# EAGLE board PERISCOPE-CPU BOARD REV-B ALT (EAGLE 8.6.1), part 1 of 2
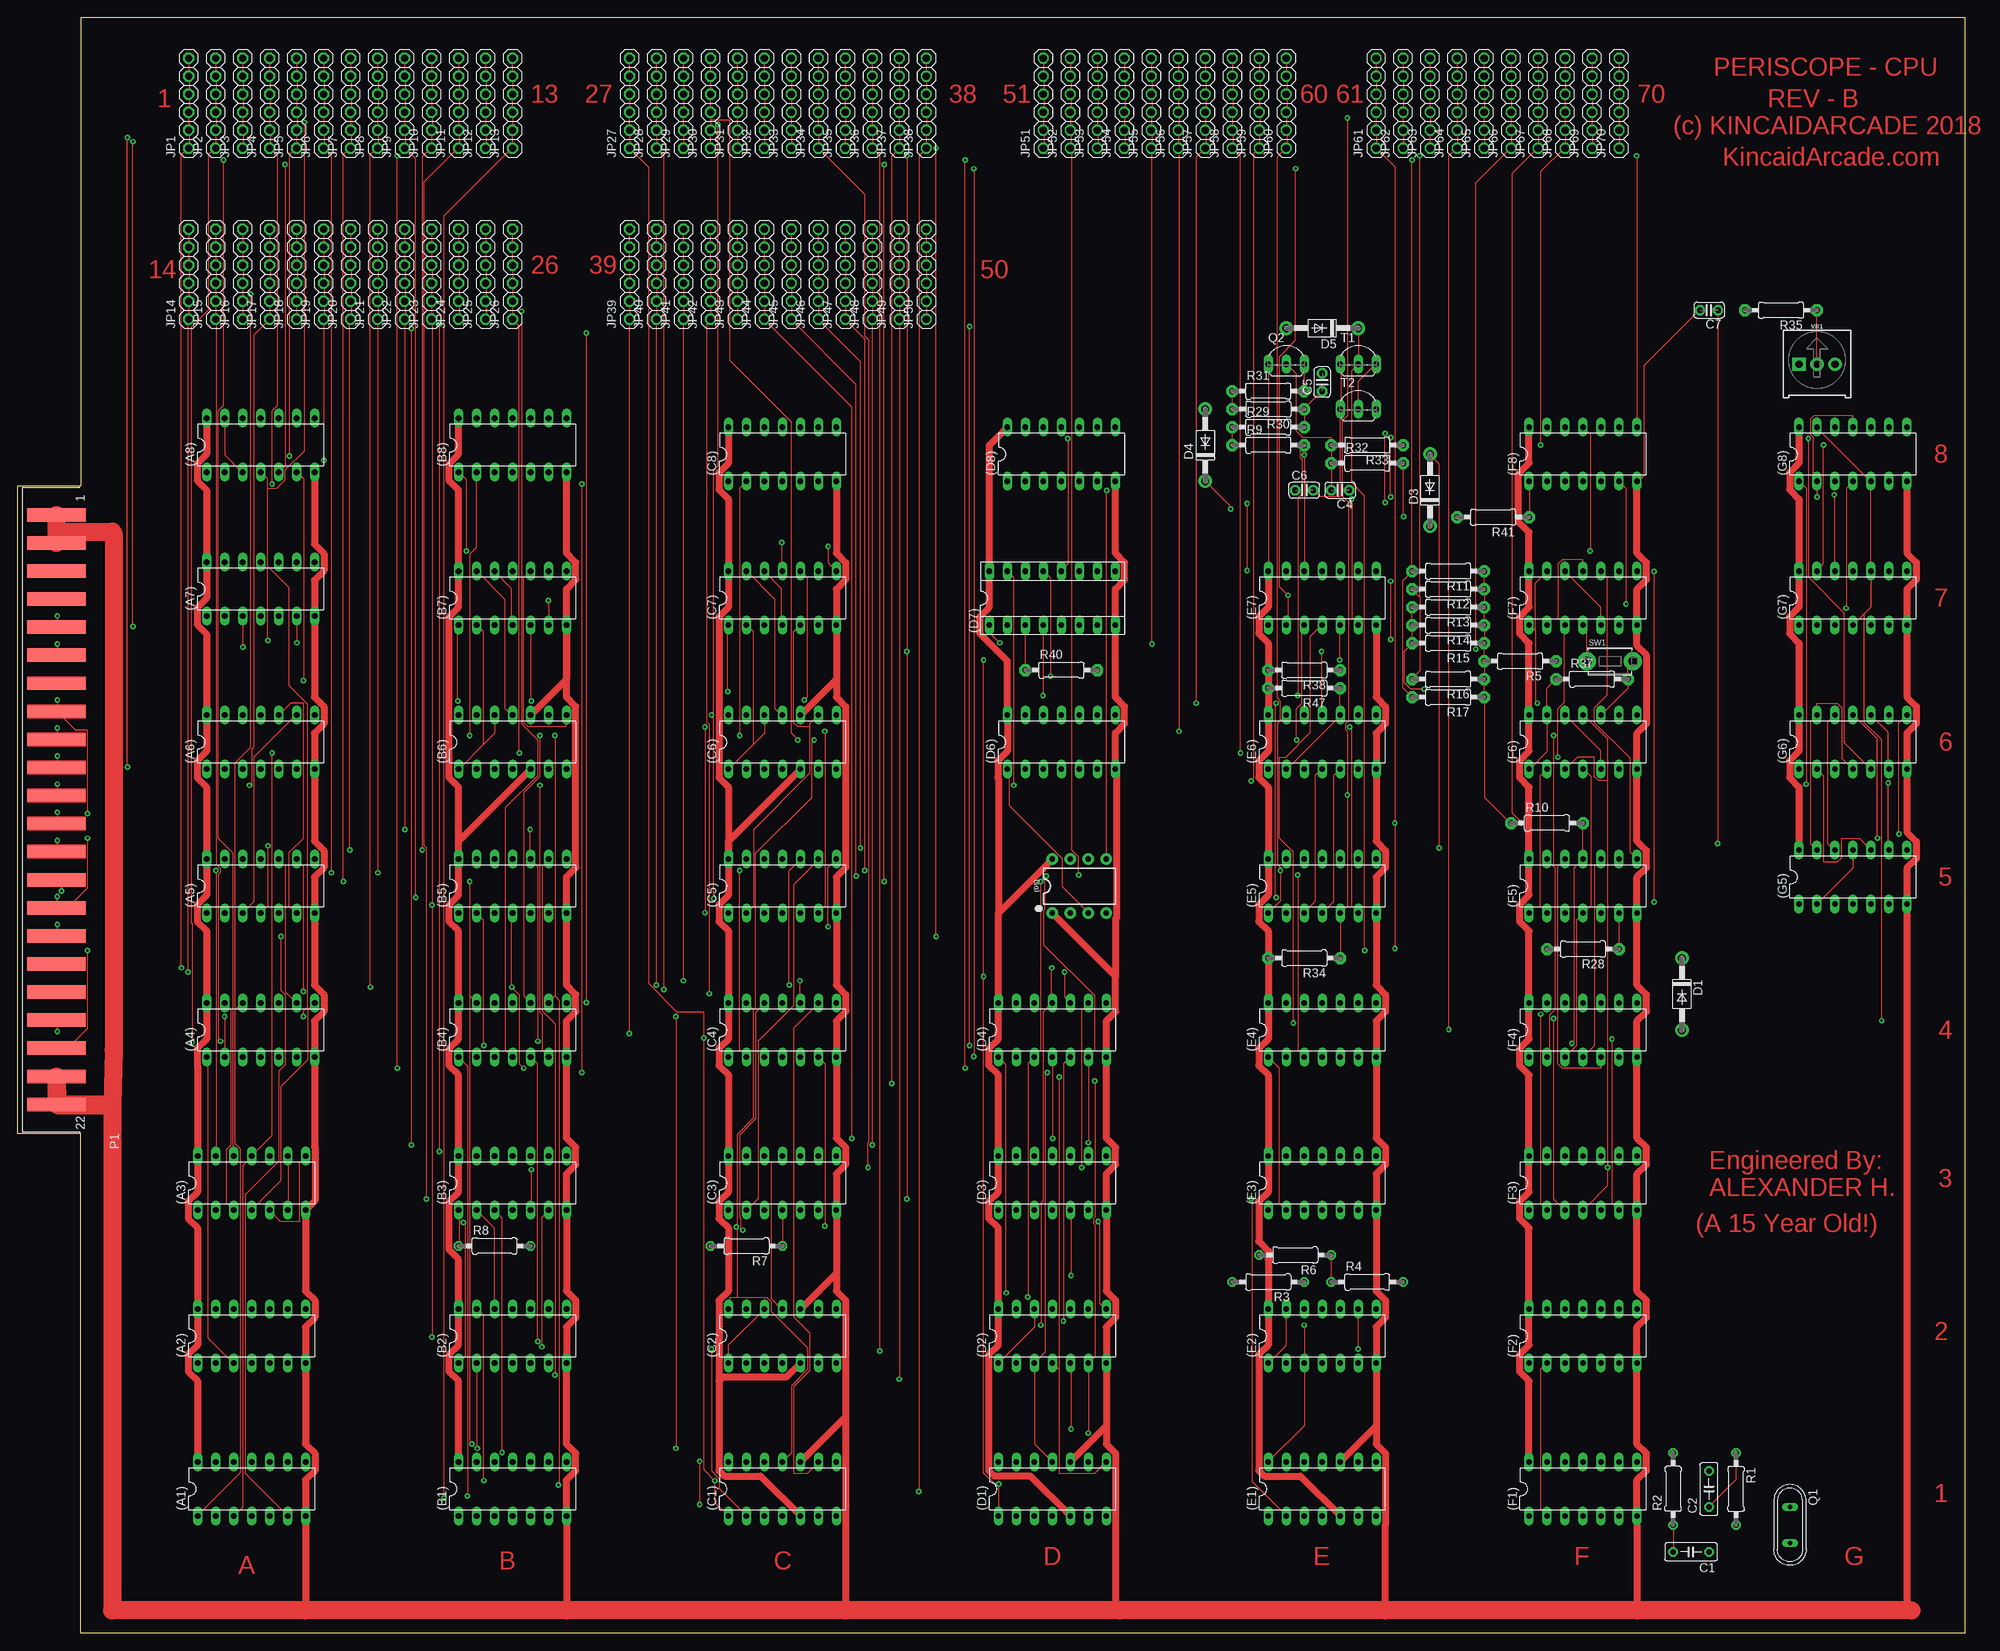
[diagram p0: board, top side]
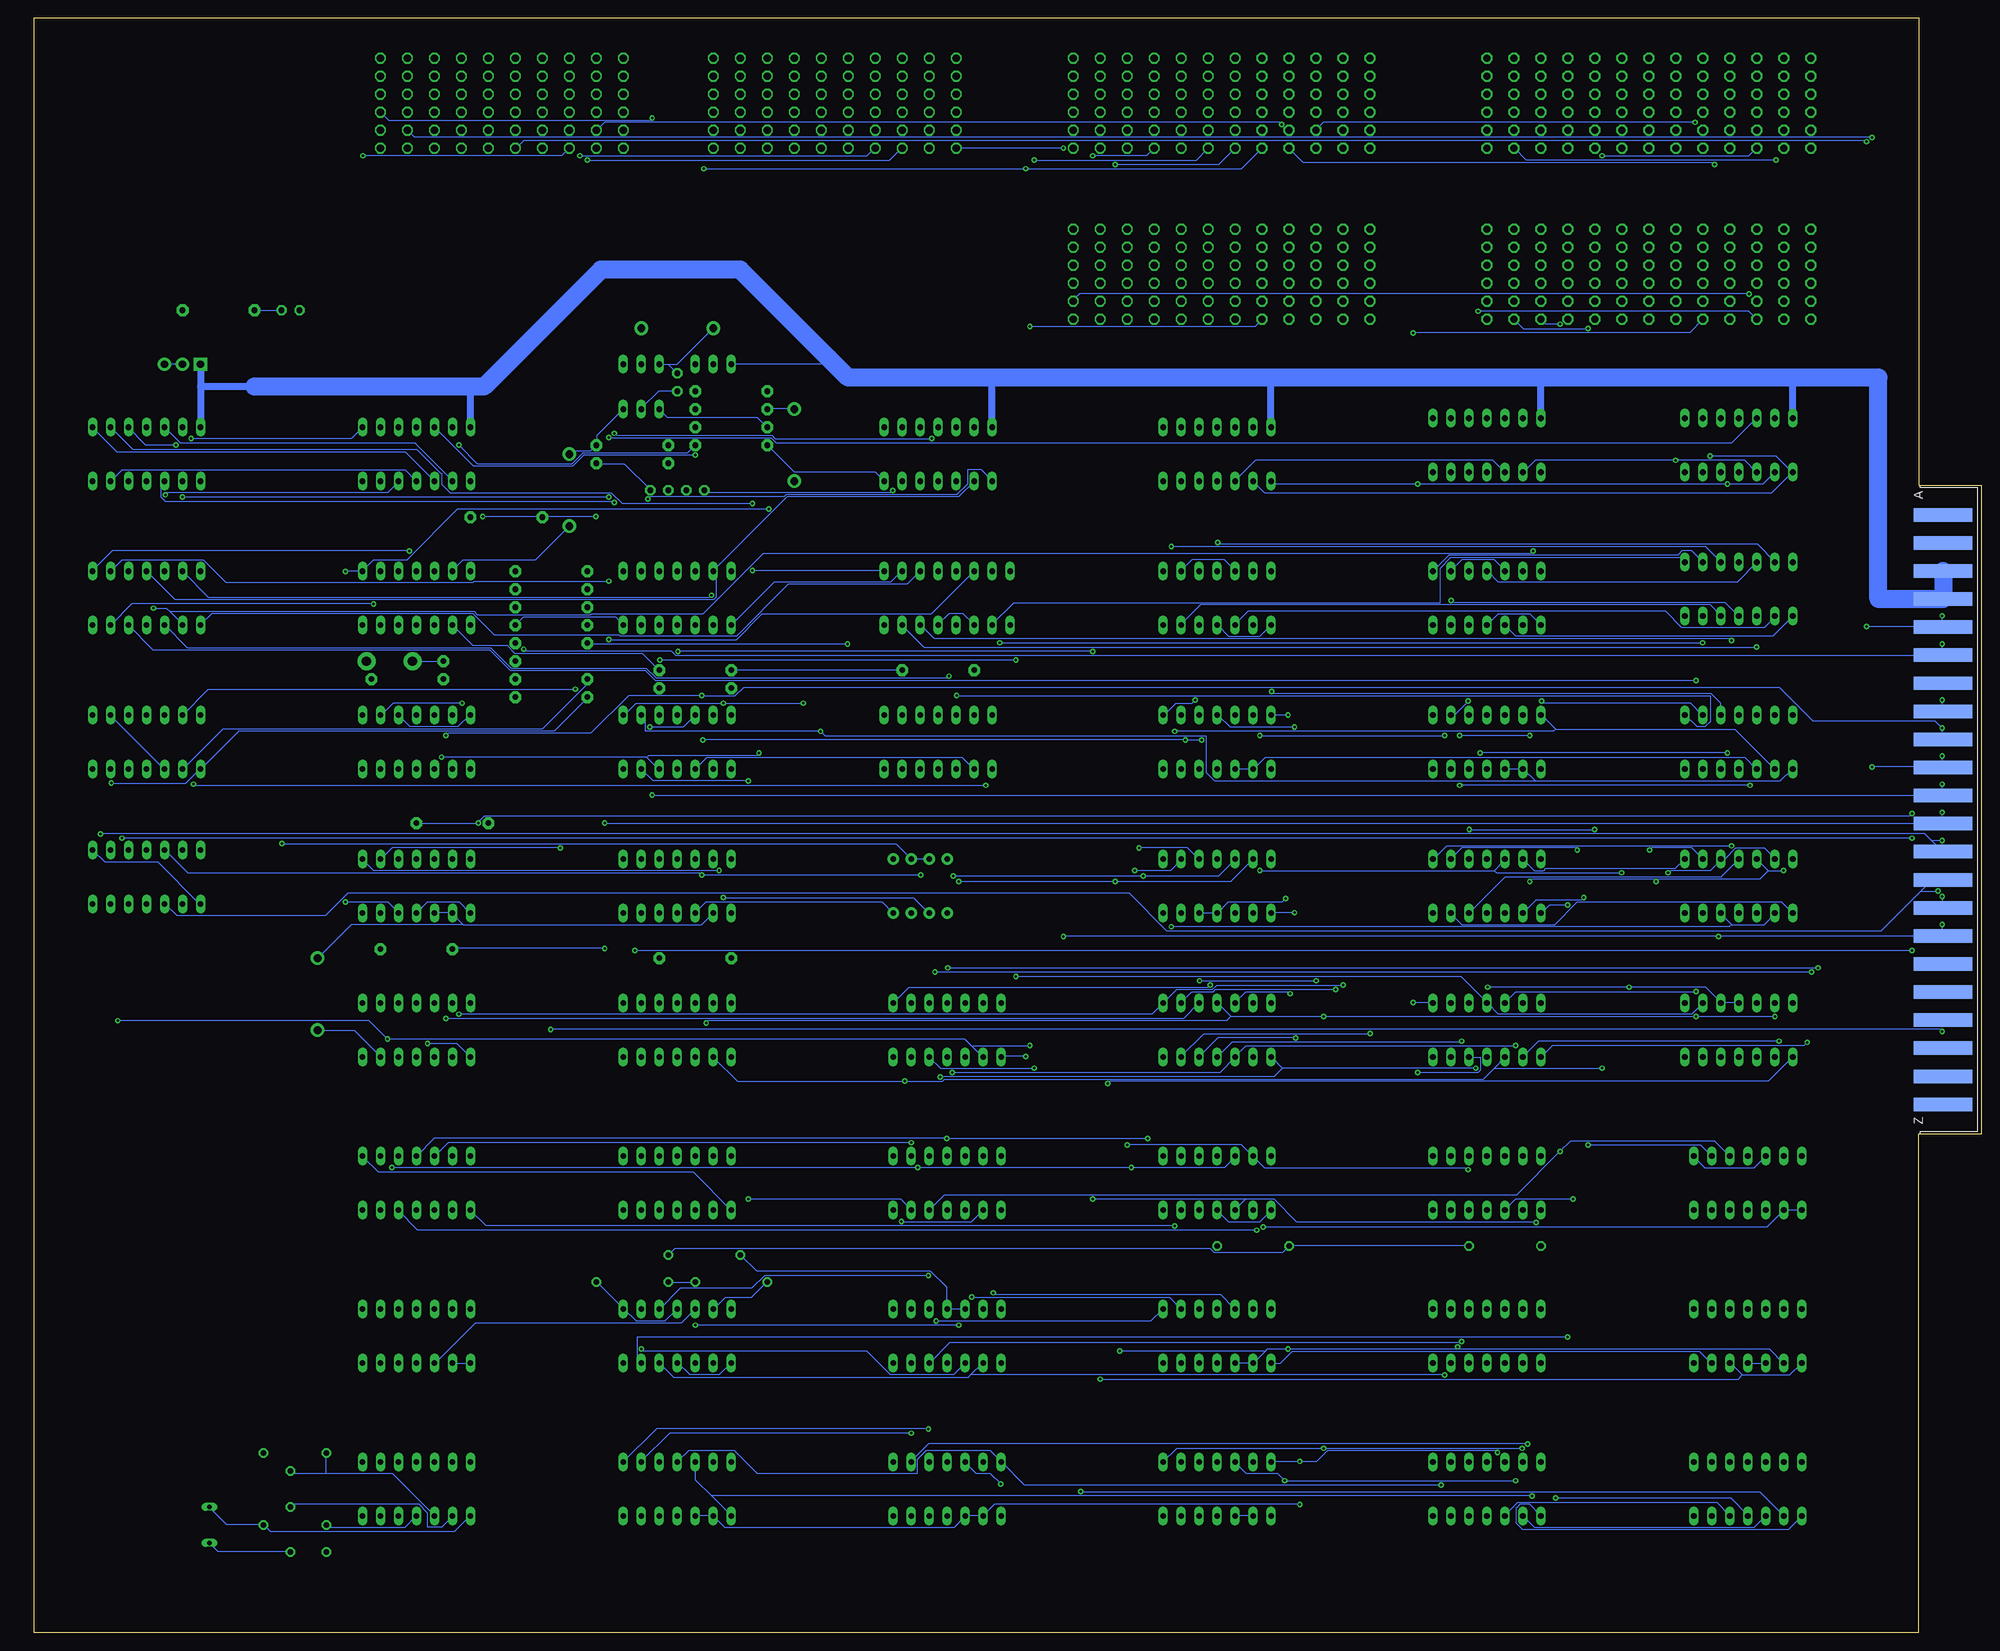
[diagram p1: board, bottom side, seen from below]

Size 274.96 x 227.97 mm. Coordinates in mm from the lower left corner, seen from the top.
Outline: 8.89,0 8.89,70.48 0,70.48 0,161.93 8.89,161.93 8.89,227.97 274.96,227.97 274.96,0 8.89,0
Copper layers (1*16): Top 0.035mm / dielectric 1.5mm / Bottom 0.035mm
Design rules "default": minimum track width 6mil, minimum drill 0.35mm, track to track 6mil, track to pad 6mil, pad to pad 6mil, via to via 6mil, smd to smd 6mil, copper to edge 40mil, drill to drill 6mil, minimum pad ring 10mil, minimum via ring 8mil, stop-mask expansion 4mil, vias tented up to drill 0mil, thermal gap 10mil

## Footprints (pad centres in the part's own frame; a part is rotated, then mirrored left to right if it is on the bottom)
DIL14 = drill 0.813 long: 1 -7.62,-3.81; 2 -5.08,-3.81; 3 -2.54,-3.81; 4 0,-3.81; 5 2.54,-3.81; 6 5.08,-3.81; 7 7.62,-3.81; 8 7.62,3.81; 9 5.08,3.81; 10 2.54,3.81; 11 0,3.81; 12 -2.54,3.81; 13 -5.08,3.81; 14 -7.62,3.81
DIP08 = drill 0.813 pad 1.626: 1 -3.81,-3.81; 2 -1.27,-3.81; 3 1.27,-3.81; 4 3.81,-3.81; 5 3.81,3.81; 6 1.27,3.81; 7 -1.27,3.81; 8 -3.81,3.81
SOCKET-16 = drill 0.813 long: 1 -8.89,-3.81; 2 -6.35,-3.81; 3 -3.81,-3.81; 4 -1.27,-3.81; 5 1.27,-3.81; 6 3.81,-3.81; 7 6.35,-3.81; 8 8.89,-3.81; 9 8.89,3.81; 10 6.35,3.81; 11 3.81,3.81; 12 1.27,3.81; 13 -1.27,3.81; 14 -3.81,3.81; 15 -6.35,3.81; 16 -8.89,3.81
C050-025X075 = drill 0.813 octagon: 1 -2.54,0; 2 2.54,0
C025-024X044 = drill 0.813 pad 1.422 octagon: 1 -1.27,0; 2 1.27,0
DO41-10 = drill 1.118 pad 1.93: A 5.08,0; C -5.08,0
1X06 = drill 1.016 octagon: 1 -6.35,0; 2 -3.81,0; 3 -1.27,0; 4 1.27,0; 5 3.81,0; 6 6.35,0
44PINEDGE = smd 1.905 x 8.255: 1 -41.605,4.826; 2 -37.643,4.826; 3 -33.68,4.826; 4 -29.718,4.826; 5 -25.756,4.826; 6 -21.793,4.826; 7 -17.831,4.826; 8 -13.868,4.826; 9 -9.906,4.826; 10 -5.944,4.826; 11 -1.981,4.826; 12 1.981,4.826; 13 5.944,4.826; 14 9.906,4.826; 15 13.868,4.826; 16 17.831,4.826; 17 21.793,4.826; 18 25.756,4.826; 19 29.718,4.826; 20 33.68,4.826; 21 37.643,4.826; 22 41.605,4.826 | smd 1.905 x 8.255 bottom: A -41.605,4.826; B -37.643,4.826; C -33.68,4.826; D -29.718,4.826; E -25.756,4.826; F -21.793,4.826; H -17.831,4.826; J -13.868,4.826; K -9.906,4.826; L -5.944,4.826; M -1.981,4.826; N 1.981,4.826; P 5.944,4.826; R 9.906,4.826; S 13.868,4.826; T 17.831,4.826; U 21.793,4.826; V 25.756,4.826; W 29.718,4.826; X 33.68,4.826; Y 37.643,4.826; Z 41.605,4.826
QS = drill 0.61 long: 1 -2.54,0; 2 2.54,0
TO92-EBC-OVAL = drill 0.813 long: B 0,-1.27; C 2.54,-1.27; E -2.54,-1.27
0207/10 = drill 0.813 octagon: 1 -5.08,0; 2 5.08,0
0207/10' = drill 0.813 pad 1.676 octagon: 1 -5.08,0; 2 5.08,0
TACT_PANA-EVQ = drill 1.3 pad 2.54: P$1 -3.25,0; P$2 3.25,0
TRIMPOT-PTH-3386U = drill 1.016 pad 1.88 square: 1 -2.54,-0.015 | drill 1.016 pad 1.88: 2 0,-0.015; 3 2.54,-0.015

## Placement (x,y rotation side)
(A1)  7404N  [DIL14]  33.02,20.32 0 top
(A2)  7402N  [DIL14]  33.02,41.91 0 top
(A3)  7400N  [DIL14]  33.02,63.5 0 top
(A4)  7410N  [DIL14]  34.29,85.09 0 top
(A5)  74S08N  [DIL14]  34.29,105.41 0 top
(A6)  7432N  [DIL14]  34.29,125.73 0 top
(A7)  7432N  [DIL14]  34.29,147.32 0 top
(A8)  74LS27N  [DIL14]  34.29,167.64 0 top
(B1)  7486N  [DIL14]  69.85,20.32 0 top
(B2)  7410N  [DIL14]  69.85,41.91 0 top
(B3)  74S74N  [DIL14]  69.85,63.5 0 top
(B4)  7404N  [DIL14]  69.85,85.09 0 top
(B5)  74LS21N  [DIL14]  69.85,105.41 0 top
(B6)  74LS93N  [DIL14]  69.85,125.73 0 top
(B7)  74S08N  [DIL14]  69.85,146.05 0 top
(B8)  7402N  [DIL14]  69.85,167.64 0 top
(C1)  74LS93N  [DIL14]  107.95,20.32 0 top
(C2)  74LS93N  [DIL14]  107.95,41.91 0 top
(C3)  74107N  [DIL14]  107.95,63.5 0 top
(C4)  7404N  [DIL14]  107.95,85.09 0 top
(C5)  74LS21N  [DIL14]  107.95,105.41 0 top
(C6)  74LS93N  [DIL14]  107.95,125.73 0 top
(C7)  74S08N  [DIL14]  107.95,146.05 0 top
(C8)  7400N  [DIL14]  107.95,166.37 0 top
(D1)  74LS93N  [DIL14]  146.05,20.32 0 top
(D2)  7430N  [DIL14]  146.05,41.91 0 top
(D3)  74LS74N  [DIL14]  146.05,63.5 0 top
(D4)  7404N  [DIL14]  146.05,85.09 0 top
(D5)  555  [DIP08]  149.86,105.41 0 top
(D6)  7404N  [DIL14]  147.32,125.73 0 top
(D7)  7448  [SOCKET-16]  146.05,146.05 0 top
(D8)  7404N  [DIL14]  147.32,166.37 0 top
(E1)  74LS93N  [DIL14]  184.15,20.32 0 top
(E2)  74LS107N  [DIL14]  184.15,41.91 0 top
(E3)  7404N  [DIL14]  184.15,63.5 0 top
(E4)  74S08N  [DIL14]  184.15,85.09 0 top
(E5)  74S08N  [DIL14]  184.15,105.41 0 top
(E6)  74S74N  [DIL14]  184.15,125.73 0 top
(E7)  7410N  [DIL14]  184.15,146.05 0 top
(F1)  7404N  [DIL14]  220.98,20.32 0 top
(F2)  7400N  [DIL14]  220.98,41.91 0 top
(F3)  7430N  [DIL14]  220.98,63.5 0 top
(F4)  7432N  [DIL14]  220.98,85.09 0 top
(F5)  7404N  [DIL14]  220.98,105.41 0 top
(F6)  74S74N  [DIL14]  220.98,125.73 0 top
(F7)  74S74N  [DIL14]  220.98,146.05 0 top
(F8)  7430N  [DIL14]  220.98,166.37 0 top
(G5)  7432N  [DIL14]  259.08,106.68 0 top
(G6)  7432N  [DIL14]  259.08,125.73 0 top
(G7)  7410N  [DIL14]  259.08,146.05 0 top
(G8)  7410N  [DIL14]  259.08,166.37 0 top
C1  100pf  [C050-025X075]  236.22,11.43 180 top
C2  .1uf  [C050-025X075]  238.76,20.32 90 top
C4  .1uf  [C025-024X044]  186.69,161.29 180 top
C5  .1uf  [C025-024X044]  184.15,176.53 90 top
C6  .01uf  [C025-024X044]  181.61,161.29 0 top
C7  100uf  [C025-024X044]  238.76,186.69 180 top
D1  1N914  [DO41-10]  234.95,90.17 270 top
D3  1N4004  [DO41-10]  199.39,161.29 90 top
D4  1N914  [DO41-10]  167.64,167.64 90 top
D5  1N914  [DO41-10]  184.15,184.15 180 top
JP1  [1X06]  24.13,215.9 90 top
JP2  [1X06]  27.94,215.9 90 top
JP3  [1X06]  31.75,215.9 90 top
JP4  [1X06]  35.56,215.9 90 top
JP5  [1X06]  39.37,215.9 90 top
JP6  [1X06]  43.18,215.9 90 top
JP7  [1X06]  46.99,215.9 90 top
JP8  [1X06]  50.8,215.9 90 top
JP9  [1X06]  54.61,215.9 90 top
JP10  [1X06]  58.42,215.9 90 top
JP11  [1X06]  62.23,215.9 90 top
JP12  [1X06]  66.04,215.9 90 top
JP13  [1X06]  69.85,215.9 90 top
JP14  [1X06]  24.13,191.77 90 top
JP15  [1X06]  27.94,191.77 90 top
JP16  [1X06]  31.75,191.77 90 top
JP17  [1X06]  35.56,191.77 90 top
JP18  [1X06]  39.37,191.77 90 top
JP19  [1X06]  43.18,191.77 90 top
JP20  [1X06]  46.99,191.77 90 top
JP21  [1X06]  50.8,191.77 90 top
JP22  [1X06]  54.61,191.77 90 top
JP23  [1X06]  58.42,191.77 90 top
JP24  [1X06]  62.23,191.77 90 top
JP25  [1X06]  66.04,191.77 90 top
JP26  [1X06]  69.85,191.77 90 top
JP27  [1X06]  86.36,215.9 90 top
JP28  [1X06]  90.17,215.9 90 top
JP29  [1X06]  93.98,215.9 90 top
JP30  [1X06]  97.79,215.9 90 top
JP31  [1X06]  101.6,215.9 90 top
JP32  [1X06]  105.41,215.9 90 top
JP33  [1X06]  109.22,215.9 90 top
JP34  [1X06]  113.03,215.9 90 top
JP35  [1X06]  116.84,215.9 90 top
JP36  [1X06]  120.65,215.9 90 top
JP37  [1X06]  124.46,215.9 90 top
JP38  [1X06]  128.27,215.9 90 top
JP39  [1X06]  86.36,191.77 90 top
JP40  [1X06]  90.17,191.77 90 top
JP41  [1X06]  93.98,191.77 90 top
JP42  [1X06]  97.79,191.77 90 top
JP43  [1X06]  101.6,191.77 90 top
JP44  [1X06]  105.41,191.77 90 top
JP45  [1X06]  109.22,191.77 90 top
JP46  [1X06]  113.03,191.77 90 top
JP47  [1X06]  116.84,191.77 90 top
JP48  [1X06]  120.65,191.77 90 top
JP49  [1X06]  124.46,191.77 90 top
JP50  [1X06]  128.27,191.77 90 top
JP51  [1X06]  144.78,215.9 90 top
JP52  [1X06]  148.59,215.9 90 top
JP53  [1X06]  152.4,215.9 90 top
JP54  [1X06]  156.21,215.9 90 top
JP55  [1X06]  160.02,215.9 90 top
JP56  [1X06]  163.83,215.9 90 top
JP57  [1X06]  167.64,215.9 90 top
JP58  [1X06]  171.45,215.9 90 top
JP59  [1X06]  175.26,215.9 90 top
JP60  [1X06]  179.07,215.9 90 top
JP61  [1X06]  191.77,215.9 90 top
JP62  [1X06]  195.58,215.9 90 top
JP63  [1X06]  199.39,215.9 90 top
JP64  [1X06]  203.2,215.9 90 top
JP65  [1X06]  207.01,215.9 90 top
JP66  [1X06]  210.82,215.9 90 top
JP67  [1X06]  214.63,215.9 90 top
JP68  [1X06]  218.44,215.9 90 top
JP69  [1X06]  222.25,215.9 90 top
JP70  [1X06]  226.06,215.9 90 top
P1  44PINEDGE  [44PINEDGE]  0.63,116.2 270 top
Q1  14.13813  [QS]  250.19,15.24 270 top
Q2  2N2907  [TO92-EBC-OVAL]  179.07,180.34 0 top
R1  330  [0207/10]  242.57,20.32 270 top
R2  330  [0207/10]  233.68,20.32 90 top
R3  1K  [0207/10]  176.53,49.53 180 top
R4  1K  [0207/10]  190.5,49.53 0 top
R5  1k  [0207/10']  212.09,137.16 180 top
R6  10k  [0207/10]  180.34,53.34 180 top
R7  1K  [0207/10]  102.87,54.61 180 top
R8  1K  [0207/10]  67.31,54.61 0 top
R9  1k  [0207/10']  176.53,167.64 0 top
R10  1k  [0207/10']  215.9,114.3 0 top
R11  1K  [0207/10']  201.93,149.86 180 top
R12  1K  [0207/10']  201.93,147.32 180 top
R13  1K  [0207/10']  201.93,144.78 180 top
R14  1K  [0207/10']  201.93,142.24 180 top
R15  1K  [0207/10']  201.93,139.7 180 top
R16  1K  [0207/10']  201.93,134.62 180 top
R17  1K  [0207/10']  201.93,132.08 180 top
R28  220  [0207/10']  220.98,96.52 180 top
R29  100  [0207/10']  176.53,170.18 0 top
R30  100  [0207/10']  176.53,172.72 180 top
R31  220  [0207/10']  176.53,175.26 0 top
R32  100  [0207/10']  190.5,165.1 0 top
R33  330  [0207/10']  190.5,167.64 180 top
R34  1K  [0207/10']  181.61,95.25 180 top
R35  220k  [0207/10']  248.92,186.69 180 top
R37  10k  [0207/10']  222.25,134.62 0 top
R38  10k  [0207/10']  181.61,135.89 180 top
R40  1K  [0207/10']  147.32,135.89 0 top
R41  1k  [0207/10']  208.28,157.48 180 top
R47  1K  [0207/10']  181.61,133.35 180 top
SW1  [TACT_PANA-EVQ]  224.79,137.16 0 top
T1  2N2222  [TO92-EBC-OVAL]  189.23,180.34 0 top
T2  2N2222  [TO92-EBC-OVAL]  189.23,173.99 0 top
VR1  1 meg  [TRIMPOT-PTH-3386U]  254,179.07 0 top

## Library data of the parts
(A1) (A2) (A3) (A4) (A5) (A6) (A7) (A8) (B1) (B2) (B3) (B4) (B5) (B6) (B7) (B8) (C1) (C2) (C3) (C4) (C5) (C6) (C7) (C8) (D1) (D2) (D3) (D4) (D6) (D8) (E1) (E2) (E3) (E4) (E5) (E6) (E7) (F1) (F2) (F3) (F4) (F5) (F6) (F7) (F8) (G5) (G6) (G7) (G8) = 74xx-us
(D5) = SparkFun-IC-Special-Function; PROD_ID: IC-09173; PROD_ID_ALT: IC-09173
(D7) = ic-package
C1 C2 R1-R4 R6-R8 = rcl
C4-C7 D1 D3-D5 JP1-JP70 Q2 R5 R9-R17 R28-R35 R37 R38 R40 R41 R47 SW1 T1 T2 = adafruit
P1 = edge-156
Q1 = special
VR1 = SparkFun-Resistors; PROD_ID: RES-09730; SF_SKU: COM-09806

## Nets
1H: (B4).1 (E1).1 (E1).12 JP2.1 JP2.2 JP2.3 JP2.4 JP2.5 JP2.6
1PSTART: (E5).5 JP70.1 JP70.2 JP70.3 JP70.4 JP70.5 JP70.6 P1.11 P1.M R34.1
1V: (B2).13 (C1).1 (C1).12 (C4).5 JP27.1 JP27.2 JP27.3 JP27.4 JP27.5 JP27.6
2H: (B4).3 (D2).6 (E1).9 (E4).2 JP3.1 JP3.2 JP3.3 JP3.4 JP3.5 JP3.6
2V: (C1).9 (C4).9 JP28.1 JP28.2 JP28.3 JP28.4 JP28.5 JP28.6
4H: (A8).2 (B4).5 (C8).1 (D2).5 (E1).8 JP4.1 JP4.2 JP4.3 JP4.4 JP4.5 JP4.6
4V: (A4).2 (A8).4 (B2).2 (C1).8 (C4).11 (E7).4 JP29.1 JP29.2 JP29.3 JP29.4 JP29.5 JP29.6
5V: R3.1 R4.1 R6.1 R7.2 R8.2
8H: (A8).1 (B4).9 (C8).2 (D1).14 (E1).11 JP5.1 JP5.2 JP5.3 JP5.4 JP5.5 JP5.6
8V: (A3).1 (A3).2 (A8).5 (C1).11 (C2).14 (C4).13 (E7).3 JP30.1 JP30.2 JP30.3 JP30.4 JP30.5 JP30.6
16H: (A4).9 (A5).10 (A5).13 (B4).11 (D1).1 (D1).12 (E7).5 JP6.1 JP6.2 JP6.3 JP6.4 JP6.5 JP6.6
16V: (A2).6 (C2).1 (C2).12 (D4).1 (E7).2 (G7).13 (G8).10 JP31.1 JP31.2 JP31.3 JP31.4 JP31.5 JP31.6
32H: (A3).13 (A5).12 (B4).13 (D1).9 JP7.1 JP7.2 JP7.3 JP7.4 JP7.5 JP7.6
32V: (C2).9 (C5).13 (D4).3 JP32.1 JP32.2 JP32.3 JP32.4 JP32.5 JP32.6
64H: (A4).10 (A4).11 (B5).4 (C4).1 (D1).8 (D2).4 JP8.1 JP8.2 JP8.3 JP8.4 JP8.5 JP8.6
64V: (C2).8 (D4).5 JP33.1 JP33.2 JP33.3 JP33.4 JP33.5 JP33.6
128H: (B5).2 (C4).3 (D1).11 (D2).3 (E2).9 JP9.1 JP9.2 JP9.3 JP9.4 JP9.5 JP9.6
128V: (C2).11 (C3).12 (D4).9 (F3).4 (F6).3 (F6).11 JP34.1 JP34.2 JP34.3 JP34.4 JP34.5 JP34.6
256H: (B5).9 (D2).2 (E2).5 JP10.1 JP10.2 JP10.3 JP10.4 JP10.5 JP10.6
256V: (B2).1 (C3).3 (E6).11 JP35.1 JP35.2 JP35.3 JP35.4 JP35.5 JP35.6
512H: (D2).1 (D2).11 (D2).12 R6.2
/1H: (B4).2 JP15.1 JP15.2 JP15.3 JP15.4 JP15.5 JP15.6
/1V: (C4).6 (F3).1 JP39.1 JP39.2 JP39.3 JP39.4 JP39.5 JP39.6
/2H: (B4).4 JP16.1 JP16.2 JP16.3 JP16.4 JP16.5 JP16.6
/2V: (C4).8 (F3).2 JP40.1 JP40.2 JP40.3 JP40.4 JP40.5 JP40.6
/4H: (B4).6 JP17.1 JP17.2 JP17.3 JP17.4 JP17.5 JP17.6
/4V: (C4).10 (F3).3 JP41.1 JP41.2 JP41.3 JP41.4 JP41.5 JP41.6
/8H: (B4).8 JP18.1 JP18.2 JP18.3 JP18.4 JP18.5 JP18.6
/8V: (C4).12 (F3).5 JP42.1 JP42.2 JP42.3 JP42.4 JP42.5 JP42.6
/16H: (A8).3 (A8).13 (B4).10 (B8).2 JP19.1 JP19.2 JP19.3 JP19.4 JP19.5 JP19.6
/16V: (D4).2 (F3).6 (G7).4 (G7).10 (G8).5 (G8).13 JP43.1 JP43.2 JP43.3 JP43.4 JP43.5 JP43.6
/32H: (A5).9 (B4).12 JP20.1 JP20.2 JP20.3 JP20.4 JP20.5 JP20.6
/32V: (D4).4 (F3).11 JP44.1 JP44.2 JP44.3 JP44.4 JP44.5 JP44.6
/64H: (B5).12 (C4).2 JP21.1 JP21.2 JP21.3 JP21.4 JP21.5 JP21.6
/64V: (C5).12 (D4).6 (F3).12 JP45.1 JP45.2 JP45.3 JP45.4 JP45.5 JP45.6
/128H: (B5).10 (C4).4 JP22.1 JP22.2 JP22.3 JP22.4 JP22.5 JP22.6
/128V: (C5).10 (D4).8 JP46.1 JP46.2 JP46.3 JP46.4 JP46.5 JP46.6
/256H: (B5).1 (E2).6 JP23.1 JP23.2 JP23.3 JP23.4 JP23.5 JP23.6
/256V: (C3).2 (C5).9 JP47.1 JP47.2 JP47.3 JP47.4 JP47.5 JP47.6
/CLK: (D4).10 JP14.1 JP14.2 JP14.3 JP14.4 JP14.5 JP14.6
/COIN: (E5).2 (F5).2 (F5).3 (F6).2 D1.C
/GAME: (E6).6 JP59.1 JP59.2 JP59.3 JP59.4 JP59.5 JP59.6
/HBLANK: (A3).6 (A3).9 JP25.1 JP25.2 JP25.3 JP25.4 JP25.5 JP25.6
/HRESET: (A3).10 (D3).5 (E2).10 JP24.1 JP24.2 JP24.3 JP24.4 JP24.5 JP24.6
/HSYNC: (A1).3 (A3).11 (B1).2 JP26.1 JP26.2 JP26.3 JP26.4 JP26.5 JP26.6
/START: (D5).2 (E6).1 (E6).8 JP57.1 JP57.2 JP57.3 JP57.4 JP57.5 JP57.6
/VBLANK: (A2).1 (A2).5 JP49.1 JP49.2 JP49.3 JP49.4 JP49.5 JP49.6
/VRESET: (B3).5 (C3).13 JP48.1 JP48.2 JP48.3 JP48.4 JP48.5 JP48.6
/VSYNC: (A1).1 (A4).12 (B1).1 JP50.1 JP50.2 JP50.3 JP50.4 JP50.5 JP50.6
A: (D7).13 (G7).3
ADDPOINT: (C5).4 (C5).5 (C6).14 JP62.1 JP62.2 JP62.3 JP62.4 JP62.5 JP62.6
ADDTENS: (A6).2 (B6).14 (C5).6
ANTENNA: D5.C P1.20 T1.B
B: (D7).12 (G8).3
BLUE: (G6).11 P1.15 P1.S
C: (D7).11 (G7).1
CLK: (D3).3 (D4).11 (E1).14 (E2).3 JP1.1 JP1.2 JP1.3 JP1.4 JP1.5 JP1.6
COIN1: (F4).1 (F5).11 JP67.1 JP67.2 JP67.3 JP67.4 JP67.5 JP67.6 P1.8 P1.J R10.2
COIN2: (F4).2 (F5).13 JP68.1 JP68.2 JP68.3 JP68.4 JP68.5 JP68.6 P1.9 P1.K R9.2
D: (D7).10 (E7).1
E: (D7).9 (G8).9
ENONES: (A5).6 (A6).10 (C7).1 (C7).4 (C7).9 (C7).12
ENTENS: (A5).3 (A6).9 (B7).1 (B7).4 (B7).9 (B7).12
F: (D7).15 (G8).1
FIRE: JP69.1 JP69.2 JP69.3 JP69.4 JP69.5 JP69.6 P1.10 P1.L
FREIGHTER: (G5).9 (G6).1 JP53.1 JP53.2 JP53.3 JP53.4 JP53.5 JP53.6 R11.2 R17.2
G: (D7).14 (G7).9
GAME: (E5).4 (E6).5 (F7).3 (F7).11 JP58.1 JP58.2 JP58.3 JP58.4 JP58.5 JP58.6
GND: (A1).7 (A2).7 (A3).7 (A4).7 (A5).7 (A6).7 (A7).7 (A8).7 (B1).7 (B2).7 (B3).7 (B4).7 (B5).7 (B6).10 (B7).7 (B8).7 (C1).10 (C2).10 (C3).7 (C4).7 (C5).7 (C6).10 (C7).7 (C8).7 (D1).10 (D2).7 (D3).7 (D4).7 (D5).1 (D6).7 (D7).8 (D8).7 (E1).10 (E2).7 (E3).7 (E4).7 (E5).7 (E6).7 (E7).7 (F1).7 (F2).7 (F3).7 (F4).7 (F5).7 (F6).7 (F7).7 (F8).7 (G5).7 (G6).7 (G7).7 (G8).7 C5.2 C6.2 C7.2 D5.A P1.1 P1.2 P1.21 P1.22 R5.2 R9.1 R10.1 R11.1 R12.1 R13.1 R14.1 R15.1 R16.1 R17.1 R29.1 T1.E T2.E
GREEN: (G5).3 P1.14 P1.R
HBLANK: (A3).5 (A3).8 (A3).12 JP12.1 JP12.2 JP12.3 JP12.4 JP12.5 JP12.6
HRESET: (B3).3 (C1).14 (D1).2 (D1).3 (D3).6 (E1).2 (E1).3 JP11.1 JP11.2 JP11.3 JP11.4 JP11.5 JP11.6
HSYNC: (A1).4 JP13.1 JP13.2 JP13.3 JP13.4 JP13.5 JP13.6
JOYDOWN: JP66.1 JP66.2 JP66.3 JP66.4 JP66.5 JP66.6 P1.6 P1.F
JOYUP: JP65.1 JP65.2 JP65.3 JP65.4 JP65.5 JP65.6 P1.5 P1.E
N$1: C1.1 Q1.2
N$2: (F1).4 C1.2 R2.1
N$3: (F1).2 (F2).1 (F2).2 C2.1 R1.1
N$4: (F1).3 C2.2 R2.2
N$5: (F1).1 Q1.1 R1.2
N$6: (E2).12 (F2).3
N$7: (E2).1 (E2).4 (E2).13 R3.2
N$8: (E2).8 (E2).11 R4.2
N$10: (A8).12 (G8).2 (G8).11
N$11: (D2).8 (D3).2
N$15: (C3).1 (C3).4 R7.1
N$16: (B3).1 R8.1
N$17: (B2).12 (B3).2
N$19: (A3).4 (A4).8
N$20: (A3).3 (A4).13
N$22: (A1).5 (B1).3
N$28: (E3).1 (F3).8
N$29: (E3).2 (E4).1
N$33: (A7).3 (D7).7
N$35: (C6).1 (C6).12 (C7).2
N$38: (F4).4 (F5).10
N$39: (F4).5 (F5).12
N$95: Q2.C R31.2
N$96: (F7).5 (F7).12
N$97: (F6).5 (F6).12
N$98: (F4).3 (F5).1 (F5).4 (F6).4
N$99: (F6).9 (F7).1 (F7).13 D3.C
N$100: (F7).4 R5.1 SW1.P$1
N$101: (F5).5 (F7).8 D4.C
N$102: (F5).6 R28.1
N$103: D4.A R30.2 R31.1
N$104: (D5).4 (E5).3 (E6).4
N$105: (F5).9 D3.A R33.1 T2.C
N$106: C4.2 Q2.B R32.1 R33.2
N$107: C5.1 R29.2 R30.1 T1.C T2.B
N$108: (E5).6 (E6).12
N$109: (D5).5 C6.1
N$112: (D6).2 (E6).3
N$114: (D5).3 (D6).1
N$115: (G6).3 (G6).9
N$116: (D5).6 (D5).7 C7.1 R35.2
N$117: (G6).6 (G6).10
N$118: R35.1 VR1.2 VR1.3
N$119: (F4).6 D1.A
N$120: (F6).1 (F6).13 R37.1
N$121: (G5).2 (G5).11
N$122: (G5).1 (G5).8
N$123: (F7).2 R38.1
N$125: (B6).1 (B6).12 (B7).2
N$126: (A5).8 (B5).13
N$127: (D8).1 (E7).6
N$128: (B6).9 (B7).5
N$129: (B6).8 (B7).10
N$130: (B6).11 (B7).13
N$131: (C5).2 (C6).9 (C7).5
N$133: (C6).8 (C7).10
N$134: (C5).1 (C6).11 (C7).13
N$135: (A7).1 (B7).3
N$136: (A7).4 (B7).6
N$137: (A7).9 (B7).8
N$138: (A7).2 (C7).3
N$139: (A7).5 (C7).6
N$140: (A7).10 (C7).8
N$141: (A7).12 (B7).11
N$142: (A7).13 (C7).11
N$143: (A6).3 (C6).2 (C6).3
N$144: (A7).6 (D7).1
N$145: (A7).8 (D7).2
N$146: (A7).11 (D7).6
N$147: (F8).2 (G8).12
N$148: (F8).3 (G8).8
N$149: (F8).4 (G8).6
N$150: (F8).5 (G7).12
N$151: (F8).6 (G7).6
N$152: (F8).11 (G7).8
N$153: (E7).12 (F8).12
N$154: (D7).3 (D7).5 R40.1
N$156: (F8).1 R41.1
N$163: (B8).3 (C8).3
N$170: (B8).1 (G7).2 (G8).4
N$174: (A8).6 (G7).5
N$177: (D8).2 (E7).13 (G7).11
N$211: (A5).11 (B5).5
N$213: (E6).2 (E6).10 R47.1
OCEAN: (E4).3 (G5).12 (G6).12 JP52.1 JP52.2 JP52.3 JP52.4 JP52.5 JP52.6
ONES: (A5).4 (B5).8
P1LED: JP61.1 JP61.2 JP61.3 JP61.4 JP61.5 JP61.6 P1.12 P1.N R28.2
Q: (E5).1 (E6).13 (F5).8 (F7).10 JP60.1 JP60.2 JP60.3 JP60.4 JP60.5 JP60.6
RED: (G6).8 P1.13 P1.P
SCORE: (F8).8 (G6).5 JP63.1 JP63.2 JP63.3 JP63.4 JP63.5 JP63.6
SCOREEN: (A6).8 (D7).4
SCOREVEN: (A5).2 (A5).5 (C5).8
SOUND: JP64.1 JP64.2 JP64.3 JP64.4 JP64.5 JP64.6 P1.19
START: (A6).1 (B6).2 (B6).3 (E6).9 JP56.1 JP56.2 JP56.3 JP56.4 JP56.5 JP56.6
SUBMARINE: (G5).10 (G6).2 JP54.1 JP54.2 JP54.3 JP54.4 JP54.5 JP54.6 R12.2 R16.2
SYNC: (A1).6 JP51.1 JP51.2 JP51.3 JP51.4 JP51.5 JP51.6 P1.16 P1.T
TENS: (A5).1 (B5).6
TORPEDO: (G5).13 (G6).4 (G6).13 JP55.1 JP55.2 JP55.3 JP55.4 JP55.5 JP55.6 R13.2 R14.2 R15.2
VBLANK: (A2).3 (A2).4 (A4).1 JP37.1 JP37.2 JP37.3 JP37.4 JP37.5 JP37.6
VCC: (A1).14 (A2).14 (A3).14 (A4).14 (A5).14 (A6).14 (A7).14 (A8).14 (B1).14 (B2).14 (B3).14 (B4).14 (B5).14 (B6).5 (B7).14 (B8).14 (C1).5 (C2).5 (C3).14 (C4).14 (C5).14 (C6).5 (C7).14 (C8).14 (D1).5 (D2).14 (D3).14 (D4).14 (D5).8 (D6).14 (D7).16 (D8).14 (E1).5 (E2).14 (E3).14 (E4).14 (E5).14 (E6).14 (E7).14 (F1).14 (F2).14 (F3).14 (F4).14 (F5).14 (F6).10 (F6).14 (F7).14 (F8).14 (G5).14 (G6).14 (G7).14 (G8).14 C4.1 P1.C P1.D Q2.E R32.2 R34.2 R37.2 R38.2 R40.2 R41.2 R47.2 SW1.P$2 VR1.1
VRESET: (A2).2 (B3).6 (C1).2 (C1).3 (C2).2 (C2).3 JP36.1 JP36.2 JP36.3 JP36.4 JP36.5 JP36.6
VSYNC: (A1).2 JP38.1 JP38.2 JP38.3 JP38.4 JP38.5 JP38.6

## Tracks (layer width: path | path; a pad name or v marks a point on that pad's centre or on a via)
1H  (via drill 0.35)
  Top 0.152: 27.99,217.17 27.99,219.61 JP2.5 27.99,219.76 27.99,222.2 JP2.6 | v24.64,83.36 24.64,100.13 24.49,100.28 24.49,184.25 26.92,186.69 26.92,208.64 27.84,209.55 JP2.1 27.99,209.55 27.99,211.99 JP2.2 27.99,212.14 27.99,214.58 JP2.3 27.99,214.73 27.99,217.17 | 27.99,217.17 JP2.4 | v63.5,19.36 63.5,80.01 (B4).1
  Bottom 0.152: 179.32,19.36 181.61,21.64 (E1).12 | 179.32,19.36 176.58,16.61 (E1).1 | (B4).1 60.6,82.91 25.09,82.91 v24.64,83.36 | v63.5,19.36 179.32,19.36
1PSTART  (via drill 0.35)
  Top 0.152: v5.59,119.79 5.59,118.26 P1.M | R34.1 186.79,95.25 186.79,101.5 (E5).5 186.79,101.65 187.71,102.56 v187.71,118.26 187.71,127.25 187.4,127.56 187.4,128.32 187.86,128.78 187.86,159.56 186.94,160.48 186.94,170.99 187.71,171.75 v187.71,213.82 | JP70.1 226.11,209.55 226.11,211.99 JP70.2 226.11,212.14 226.11,214.58 JP70.3 226.11,214.73 226.11,217.17 | 226.11,217.17 226.11,219.61 JP70.5 226.11,219.76 226.11,222.2 JP70.6 | 226.11,217.17 JP70.4
  Bottom 0.152: 5.59,118.26 v5.59,119.79 | v187.71,213.82 188.01,213.51 224.89,213.51 225.96,214.58 JP70.3 | v187.71,118.26 5.59,118.26 | 5.59,118.26 P1.M
1V  (via drill 0.35)
  Top 0.152: JP27.6 JP27.5 JP27.4 JP27.3 JP27.2 JP27.1 89.1,206.81 89.1,91.59 93.07,87.63 96.88,87.63 v96.88,83.97 96.88,23.01 v98.4,21.49 98.4,18.44 (C1).1 | v65.79,21.49 65.79,44.81 64.87,45.72 (B2).13
  Bottom 0.152: (C1).12 105.41,24.08 103.89,22.55 99.47,22.55 v98.4,21.49 v65.79,21.49 | v96.88,83.97 107.85,83.97 110.44,81.38 (C4).5
2H  (via drill 0.35)
  Top 0.152: JP3.1 31.8,209.55 31.8,211.99 JP3.2 31.8,212.14 31.8,214.58 JP3.3 31.8,214.73 31.8,217.17 | 31.8,217.17 31.8,219.61 JP3.5 31.8,219.76 31.8,222.2 JP3.6 | 31.8,217.17 JP3.4 | v152.04,77.88 152.04,58.67 151.89,58.52 151.89,57.76 152.04,57.61 152.04,39.01 (D2).6 v151.13,28.19 | v53.59,79.7 v53.59,208.48
  Bottom 0.152: 68.83,79.7 70.36,78.18 146.41,78.18 146.71,77.88 v152.04,77.88 175.67,77.88 (E4).2 | 68.83,79.7 67.31,81.23 (B4).3 | v151.13,28.19 185.27,28.19 189.23,24.23 (E1).9 | v53.59,208.48 32.87,208.48 31.8,209.55 JP3.1 | 68.83,79.7 v53.59,79.7
2V  (via drill 0.35)
  Top 0.152: JP28.6 JP28.5 JP28.4 JP28.3 JP28.2 JP28.1 91.24,208.48 v91.24,90.83 | (C1).9 113.03,24.08 111.51,22.55 109.52,22.55 109.52,34.75 111.81,37.03 111.81,42.37 109.52,44.65 109.52,85.34 113.03,88.85 (C4).9
  Bottom 0.152: v91.24,90.83 108.15,90.83 108.46,90.53 111.51,90.53 113.03,89 (C4).9
4H  (via drill 0.35)
  Top 0.152: 35.61,209.55 35.61,211.99 JP4.2 35.61,212.14 35.61,214.58 JP4.3 35.61,214.73 35.61,217.17 | 35.61,217.17 35.61,219.61 JP4.5 35.61,219.76 35.61,222.2 JP4.6 | 35.61,217.17 JP4.4 | 35.61,209.55 36.68,208.48 36.68,173.28 35.92,172.52 v35.92,162.15 | 35.61,209.55 JP4.1 | v73.41,41.15 73.41,80.31 72.49,81.23 (B4).5 | v148.69,28.8 148.69,38.1 (D2).5 | v79.65,79.1 v79.65,162.15
  Bottom 0.152: (C8).1 99.92,162.15 v79.65,162.15 v35.92,162.15 30.89,162.15 (A8).2 | v73.41,41.15 73.56,41 145.64,41 148.54,38.1 (D2).5 | (E1).8 187.1,28.8 v148.69,28.8 | v79.65,79.1 71.12,79.1 70.81,79.4 70.81,81.23 72.34,81.23 (B4).5
4V  (via drill 0.35)
  Top 0.152: v64.87,26.06 64.87,38.1 (B2).2 | JP29.1 JP29.2 JP29.3 JP29.4 JP29.5 JP29.6 | v29.21,87.02 (A4).2 | v180.09,86.11 180.09,110.19 178.1,112.17 178.1,123.6 179.02,123.6 182.52,127.1 182.52,140.66 184.05,142.19 (E7).4 | 35.31,161.54 35.31,150.57 38.35,147.52 38.35,133.66 40.95,131.06 40.95,88.39 40.34,87.78 v40.34,87.02 | 35.31,161.54 35.31,162.92 34.39,163.83 (A8).4 | v40.49,213.21 40.49,166.88 37.74,164.13 37.74,162.76 36.52,161.54 35.31,161.54 | v92.91,87.02 v92.91,26.06
  Bottom 0.152: v64.87,26.06 v92.91,26.06 113.64,26.06 (C1).8 | 106.02,87.02 v92.91,87.02 v40.34,87.02 v29.21,87.02 | 106.02,87.02 107.85,88.85 (C4).11 | v180.09,86.11 179.78,86.41 106.63,86.41 106.02,87.02 | v40.49,213.21 92.91,213.21 93.98,212.14 JP29.2
5V
  Top 0.152: R4.1 R6.1
  Bottom 0.152: R4.1 R3.1 | R8.2 72.49,54.71 97.79,54.71 R7.2 97.79,54.56 98.7,53.65 108.31,53.65 108.91,54.25 184.51,54.25 R6.1
8H  (via drill 0.35)
  Top 0.152: 39.42,217.17 39.42,219.61 JP5.5 39.42,219.76 39.42,222.2 JP5.6 | v38.35,166.12 38.35,208.64 39.27,209.55 JP5.1 39.42,209.55 39.42,211.99 JP5.2 39.42,212.14 39.42,214.58 JP5.3 39.42,214.73 39.42,217.17 | 39.42,217.17 JP5.4 | 75.84,89.92 74.93,89 (B4).9 | v75.84,126.64 75.84,89.92 | v101.91,126.64 101.91,161.54 102.82,162.46 (C8).2 | v76.3,20.88 76.45,21.03 76.45,89.31 75.84,89.92
  Bottom 0.152: 26.77,163.83 29.06,166.12 v38.35,166.12 | (E1).11 182.52,25.76 176.12,25.76 172.92,22.55 150.22,22.55 150.22,24.54 149,25.76 140,25.76 138.48,24.23 (D1).14 138.33,24.08 135.13,20.88 v76.3,20.88 | v101.91,126.64 v75.84,126.64 | 26.77,163.83 29.67,160.93 101.3,160.93 102.82,162.46 (C8).2 | 26.77,163.83 (A8).1
8V  (via drill 0.35)
  Top 0.152: JP30.6 JP30.5 JP30.4 JP30.3 97.79,213.51 | 97.79,213.51 JP30.2 JP30.1 | (A8).5 37.74,164.74 v37.74,207.26 | 101.6,47.4 100.53,47.4 100.53,45.87 100.38,45.72 (C2).14 | 101.6,47.4 105.72,47.4 106.32,46.79 106.32,45.41 111.51,40.23 111.51,37.19 109.22,34.9 109.22,25.45 108,24.23 (C1).11 | 103.89,87.94 102.97,88.85 (C4).13 | 103.89,87.94 103.89,72.7 101.6,70.41 101.6,57.3 | 101.6,47.4 101.6,57.3 | v180.54,126.03 180.54,130.45 181.31,131.22 181.31,141.88 181.61,142.19 (E7).3 | v112.42,126.03 112.12,125.73 112.12,117.96 104.19,110.03 104.19,88.24 103.89,87.94 | 101.6,57.3 v101.45,57.3 | 97.79,213.51 100.53,213.51 100.53,179.53 109.22,170.84 109.22,126.95 v110.13,126.03
  Bottom 0.152: v37.74,207.26 38.05,207.57 95.81,207.57 JP30.1 | (A3).1 25.4,59.74 27.84,59.74 (A3).2 27.99,59.59 30.28,57.3 v101.45,57.3 | v180.54,126.03 v112.42,126.03 v110.13,126.03
16H  (via drill 0.35)
  Top 0.152: 43.23,209.55 43.23,211.99 JP6.2 43.23,212.14 43.23,214.58 JP6.3 43.23,214.73 43.23,217.17 | 43.23,217.17 43.23,219.61 JP6.5 43.23,219.76 43.23,222.2 JP6.6 | 43.23,217.17 JP6.4 | (A4).9 37.74,90.53 37.74,108.2 36.83,109.12 (A5).10 | 43.23,209.55 44.3,208.48 v44.3,107.29 | 43.23,209.55 JP6.1 | (D1).1 138.48,16.61 v138.48,21.03 137.87,21.03 136.35,22.55 v136.35,92.66 v136.35,137.31 | v186.64,137.31 186.64,142.19 (E7).5
  Bottom 0.152: (A5).13 29.21,109.27 30.73,110.8 34.7,110.8 36.22,109.27 36.83,109.27 (A5).10 36.83,109.12 38.35,107.59 43.99,107.59 v44.3,107.29 | (A4).9 40.95,87.33 68.22,87.33 69.75,88.85 (B4).11 69.9,89 73.56,92.66 v136.35,92.66 | v138.48,21.03 140,22.55 141.99,22.55 143.51,24.08 (D1).12 | v136.35,137.31 v186.64,137.31
16V  (via drill 0.35)
  Top 0.152: (C2).12 100.38,40.69 100.38,38.1 (C2).1 | (D4).1 139.55,80.16 v139.55,48.01 | JP31.1 JP31.2 JP31.3 JP31.4 JP31.5 JP31.6 | (E7).2 179.32,142.49 v179.32,146.46 178.1,147.68 178.1,180.14 180.39,182.42 v180.39,206.65 | v254.91,167.64 254.91,150.88 254,149.96 (G7).13 | v134.98,206.65 v134.98,81.38
  Bottom 0.152: (C2).1 99.01,38.1 97.33,39.78 39.88,39.78 38.2,38.1 (A2).6 | v139.55,48.01 139.24,47.7 107.39,47.7 (C2).12 | v179.32,146.46 179.63,146.15 250.34,146.15 254,149.81 (G7).13 | v254.91,167.64 259.18,167.64 261.62,170.08 (G8).10 | JP31.1 104.5,206.65 v134.98,206.65 v180.39,206.65 | v134.98,81.38 138.33,81.38 (D4).1
32H  (via drill 0.35)
  Top 0.152: 47.04,217.17 47.04,219.61 JP7.5 47.04,219.76 47.04,222.2 JP7.6 | 47.04,217.17 47.04,214.73 JP7.3 47.04,214.58 47.04,212.14 JP7.2 47.04,211.99 47.04,209.55 JP7.1 46.89,209.55 45.97,208.64 v45.97,106.07 | 47.04,217.17 JP7.4 | v27.99,107.59 27.99,67.36 (A3).13 | 63.81,89.92 64.72,89 (B4).13 | v63.81,106.07 63.81,89.92 | v64.11,26.67 63.81,26.97 63.81,89.92
  Bottom 0.152: 30.12,107.59 v27.99,107.59 | (A5).12 30.12,107.59 | v63.81,106.07 63.5,106.38 45.97,106.38 | 45.97,106.38 31.34,106.38 30.12,107.59 | v64.11,26.67 148.69,26.67 151.13,24.23 (D1).9 | 45.97,106.38 v45.97,106.07
32V  (via drill 0.35)
  Top 0.152: JP32.1 JP32.2 JP32.3 JP32.4 JP32.5 JP32.6 | v142.6,47.4 142.6,80.31 143.51,81.23 (D4).3 143.51,81.38 144.42,82.3 v144.42,106.07 | v122.33,106.07 v122.33,207.26
  Bottom 0.152: (C2).9 114.71,47.4 v142.6,47.4 | (C5).13 106.02,106.07 v122.33,106.07 v144.42,106.07 | JP32.1 107.7,207.26 v122.33,207.26
64H  (via drill 0.35)
  Top 0.152: 147.01,37.19 147.01,22.55 152.04,22.55 153.57,24.08 (D1).8 | 147.01,37.19 146.1,38.1 (D2).4 | 50.85,217.17 50.85,219.61 JP8.5 50.85,219.76 50.85,222.2 JP8.6 | 50.85,217.17 50.85,214.73 JP8.3 50.85,214.58 50.85,212.14 JP8.2 50.85,211.99 50.85,209.55 JP8.1 50.7,209.55 49.78,208.64 v49.78,91.14 | 50.85,217.17 JP8.4 | (B5).4 69.75,101.5 v69.75,91.14 70.81,90.07 70.81,80.31 v71.42,79.7 | v147.01,78.49 147.01,37.19
  Bottom 0.152: 36.83,89 34.39,89 (A4).11 | v69.75,91.14 v49.78,91.14 38.96,91.14 36.83,89 | 36.83,89 (A4).10 | 98.7,79.7 100.23,81.23 (C4).1 | v71.42,79.7 98.7,79.7 | v147.01,78.49 99.92,78.49 98.7,79.7
64V  (via drill 0.35)
  Top 0.152: JP33.1 JP33.2 JP33.3 JP33.4 JP33.5 JP33.6 | v147.62,44.04 147.62,80.31 (D4).5 | v133.76,79.7 v133.76,207.87
  Bottom 0.152: v147.62,44.04 117.3,44.04 115.62,45.72 (C2).8 | JP33.1 110.9,207.87 v133.76,207.87 | v133.76,79.7 147.01,79.7 (D4).5
128H  (via drill 0.35)
  Top 0.152: (D1).11 143.51,26.67 (D2).3 145.03,39.62 145.03,78.79 v145.34,79.1 | v189.23,40.08 (E2).9 | 54.66,209.55 54.66,211.99 JP9.2 54.66,212.14 54.66,214.58 JP9.3 54.66,214.73 54.66,217.17 | 54.66,217.17 54.66,219.61 JP9.5 54.66,219.76 54.66,222.2 JP9.6 | 54.66,217.17 JP9.4 | (B5).2 65.79,100.58 v65.79,82.91 | 54.66,209.55 56.19,208.03 v56.19,103.78 | 54.66,209.55 JP9.1
  Bottom 0.152: v189.23,40.08 188.92,39.78 157.38,39.78 154.03,36.42 145.19,36.42 (D2).3 | v65.79,82.91 103.89,82.91 105.41,81.38 (C4).3 105.41,81.23 107.54,79.1 v145.34,79.1 | v56.19,103.78 56.49,103.48 62.89,103.48 (B5).2
128V  (via drill 0.35)
  Top 0.152: 224.43,120.24 224.43,126.19 221.08,129.54 (F6).11 | 224.43,120.24 v224.43,65.68 224.43,63.09 221.08,59.74 (F3).4 | 224.43,120.24 223.22,120.24 222.61,120.85 222.61,123.6 220.17,123.6 218.49,121.92 (F6).3 | JP34.6 JP34.5 JP34.4 JP34.3 JP34.2 JP34.1 119.58,203 119.58,183.03 120.19,182.42 120.19,69.34 120.04,69.19 v120.04,65.68 | (C2).11 107.85,45.72 106.32,47.24 106.32,66.29 105.41,67.21 (C3).12 | v150.22,65.68 150.22,87.94 151.13,88.85 (D4).9
  Bottom 0.152: (C3).12 105.41,67.21 106.93,65.68 v120.04,65.68 v150.22,65.68 v224.43,65.68
256H  (via drill 0.35)
  Top 0.152: 58.47,217.17 58.47,219.61 JP10.5 58.47,219.76 58.47,222.2 JP10.6 | v57.1,110.49 57.1,208.33 58.32,209.55 JP10.1 58.47,209.55 58.47,211.99 JP10.2 58.47,212.14 58.47,214.58 JP10.3 58.47,214.73 58.47,217.17 | 58.47,217.17 JP10.4 | v75.84,36.42 75.84,85.95 74.02,87.78 74.02,108.2 74.93,109.12 (B5).9
  Bottom 0.152: 142.75,36.42 143.05,36.12 184.66,36.12 186.64,38.1 (E2).5 | 142.75,36.42 141.07,38.1 (D2).2 | v57.1,110.49 57.4,110.8 73.41,110.8 74.93,109.27 (B5).9 | v75.84,36.42 142.75,36.42
256V  (via drill 0.35)
  Top 0.152: v62.89,57.91 63.19,57.61 63.19,39.01 62.28,38.1 (B2).1 | JP35.6 JP35.5 JP35.4 JP35.3 JP35.2 JP35.1 | v184.05,138.53 184.05,129.54 (E6).11 | v125.53,208.48 v125.53,138.53 v125.53,61.27
  Bottom 0.152: v62.89,57.91 63.04,58.06 96.72,58.06 99.92,61.27 103.89,61.27 | 103.89,61.27 105.41,59.74 (C3).3 | v125.53,138.53 v184.05,138.53 | v125.53,208.48 117.91,208.48 JP35.1 | v125.53,61.27 103.89,61.27
512H
  Top 0.152: (D2).12 143.51,43.13 138.48,38.1 (D2).1
  Bottom 0.152: (D2).12 (D2).11 146.1,45.72 146.1,48.77 148.39,51.05 172.92,51.05 175.21,53.34 R6.2
/1H  (via drill 0.35)
  Top 0.152: 27.99,190.5 27.99,192.94 JP15.4 27.99,193.09 27.99,195.53 JP15.5 27.99,195.68 27.99,198.12 JP15.6 | v28.6,83.52 28.3,83.82 28.3,106.98 28.6,107.29 28.6,107.9 27.99,108.51 27.99,185.32 JP15.1 27.99,185.47 27.99,187.91 JP15.2 27.99,188.06 27.99,190.5 | 27.99,190.5 JP15.3
  Bottom 0.152: v28.6,83.52 62.59,83.52 64.72,81.38 (B4).2
/1V  (via drill 0.35)
  Top 0.152: JP39.6 JP39.5 JP39.4 JP39.3 JP39.2 JP39.1 v86.36,84.58 | v113.94,57.46 113.94,80.31 113.03,81.23 (C4).6
  Bottom 0.152: v113.94,57.46 211.18,57.46 213.31,59.59 (F3).1 | v86.36,84.58 109.83,84.58 113.03,81.38 (C4).6
/2H  (via drill 0.35)
  Top 0.152: 31.8,190.5 31.8,192.94 JP16.4 31.8,193.09 31.8,195.53 JP16.5 31.8,195.68 31.8,198.12 JP16.6 | (B4).4 68.83,82.3 68.83,116.43 73.41,121.01 73.41,126.03 71.12,128.32 v71.12,186.54 | JP16.1 31.8,185.47 31.8,187.91 JP16.2 31.8,188.06 31.8,190.5 | 31.8,190.5 JP16.3
  Bottom 0.152: v71.12,186.54 32.87,186.54 JP16.1
/2V  (via drill 0.35)
  Top 0.152: JP40.6 JP40.5 JP40.4 JP40.3 JP40.2 JP40.1 v90.17,91.44 | v214.99,87.33 214.99,60.66 215.9,59.74 (F3).2
  Bottom 0.152: v214.99,87.33 117.14,87.33 (C4).8 113.64,90.83 108.61,90.83 108,91.44 v90.17,91.44
/4H  (via drill 0.35)
  Top 0.152: 35.61,190.5 35.61,192.94 JP17.4 35.61,193.09 35.61,195.53 JP17.5 35.61,195.68 35.61,198.12 JP17.6 | v73.71,119.63 73.71,87.63 74.02,87.33 74.02,82.3 74.93,81.38 (B4).6 | v32.72,119.63 33.02,119.94 33.02,124.66 33.33,124.97 33.33,183.19 JP17.1 35.61,185.47 35.61,187.91 JP17.2 35.61,188.06 35.61,190.5 | 35.61,190.5 JP17.3
  Bottom 0.152: v32.72,119.63 v73.71,119.63
/4V  (via drill 0.35)
  Top 0.152: JP41.6 JP41.5 JP41.4 JP41.3 JP41.2 JP41.1 v93.98,92.05 | v216.81,86.72 216.81,61.27 218.34,59.74 (F3).3 | v110.44,92.05 110.44,89 (C4).10
  Bottom 0.152: v216.81,86.72 112.72,86.72 110.59,88.85 (C4).10 | v110.44,92.05 v93.98,92.05
/8H  (via drill 0.35)
  Top 0.152: 39.42,190.5 39.42,192.94 JP18.4 39.42,193.09 39.42,195.53 JP18.5 39.42,195.68 39.42,198.12 JP18.6 | v80.26,183.49 v80.26,89 | JP18.1 39.42,185.47 39.42,187.91 JP18.2 39.42,188.06 39.42,190.5 | 39.42,190.5 JP18.3
  Bottom 0.152: v80.26,89 77.52,89 (B4).8 | v80.26,183.49 41.25,183.49 39.42,185.32 JP18.1
/8V  (via drill 0.35)
  Top 0.152: JP42.6 JP42.5 JP42.4 JP42.3 JP42.2 JP42.1 97.79,185.32 97.33,184.86 97.33,128.47 97.64,128.17 v97.64,90.22 | v102.36,56.84 102.06,57.15 102.06,58.52 101.91,58.67 101.91,70.26 104.19,72.54 104.19,87.63 105.41,88.85 (C4).12
  Bottom 0.152: v102.36,56.84 220.78,56.84 223.52,59.59 (F3).5 | v97.64,90.22 97.94,90.53 103.89,90.53 105.41,89 (C4).12
/16H  (via drill 0.35)
  Top 0.152: 43.23,190.5 43.23,192.94 JP19.4 43.23,193.09 43.23,195.53 JP19.5 43.23,195.68 43.23,198.12 JP19.6 | 43.23,190.5 43.23,188.06 JP19.2 43.23,187.91 43.23,185.47 JP19.1 43.23,185.32 v43.23,165.51 | 43.23,190.5 JP19.3 | (A8).13 29.21,166.27 31.65,163.83 (A8).3 | v73.71,126.64 73.71,120.85 71.42,118.57 71.42,89.92 72.34,89 (B4).10 | v63.81,126.64 63.81,152.25 64.72,153.16 64.72,163.83 (B8).2
  Bottom 0.152: (B8).2 64.72,163.83 63.04,165.51 v43.23,165.51 33.48,165.51 31.8,163.83 (A8).3 | v63.81,126.64 v73.71,126.64
/16V  (via drill 0.35)
  Top 0.152: 260.71,143.87 261.62,144.78 (G7).10 261.62,162.46 | 260.71,143.87 (G7).4 | 261.62,162.46 254,170.08 (G8).13 | 261.62,162.46 (G8).5 | JP43.1 JP43.2 JP43.3 JP43.4 JP43.5 JP43.6 | v225.04,83.82 225.04,60.66 225.96,59.74 (F3).6 | v134.37,82.91 v134.37,184.4 | 260.71,143.87 260.71,128.47 263.14,126.03 v263.14,86.41
  Bottom 0.152: (D4).2 142.6,82.91 | 142.6,82.91 143.51,83.82 v225.04,83.82 227.63,86.41 v263.14,86.41 | v134.37,184.4 102.51,184.4 101.6,185.32 JP43.1 | 142.6,82.91 v134.37,82.91
/32H  (via drill 0.35)
  Top 0.152: 47.04,190.5 47.04,192.94 JP20.4 47.04,193.09 47.04,195.53 JP20.5 47.04,195.68 47.04,198.12 JP20.6 | 47.04,190.5 47.04,188.06 JP20.2 47.04,187.91 47.04,185.47 JP20.1 46.89,185.32 v46.89,110.49 | 47.04,190.5 JP20.3 | v40.34,90.53 40.34,108.2 39.42,109.12 (A5).9
  Bottom 0.152: v40.34,90.53 65.79,90.53 67.31,89 (B4).12 | v46.89,110.49 46.58,110.8 40.95,110.8 (A5).9
/32V  (via drill 0.35)
  Top 0.152: JP44.6 JP44.5 JP44.4 JP44.3 JP44.2 JP44.1 105.41,185.32 117.75,172.97 v117.75,69.8 | v146.1,69.8 146.1,81.23 (D4).4
  Bottom 0.152: (F3).11 218.49,69.8 v146.1,69.8 v117.75,69.8
/64H  (via drill 0.35)
  Top 0.152: 50.85,190.5 50.85,192.94 JP21.4 50.85,193.09 50.85,195.53 JP21.5 50.85,195.68 50.85,198.12 JP21.6 | 50.85,190.5 50.85,188.06 JP21.2 50.85,187.91 50.85,185.47 JP21.1 50.85,185.32 v50.85,107.29 | 50.85,190.5 JP21.3 | v101.91,107.59 101.91,82.3 102.82,81.38 (C4).2
  Bottom 0.152: 68.83,107.59 67.31,109.12 (B5).12 | v101.91,107.59 68.83,107.59 | v50.85,107.29 68.53,107.29 68.83,107.59
/64V  (via drill 0.35)
  Top 0.152: JP45.6 JP45.5 JP45.4 JP45.3 JP45.2 JP45.1 109.22,185.32 118.36,176.17 v118.36,106.83 | v145.19,106.83 145.03,106.68 145.03,102.11 144.88,101.96 144.88,97.08 152.04,89.92 152.04,82.3 151.13,81.38 (D4).6 v151.13,69.19
  Bottom 0.152: v145.19,106.83 v118.36,106.83 107.7,106.83 105.41,109.12 (C5).12 | v151.13,69.19 216.51,69.19 218.34,67.36 (F3).12
/128H  (via drill 0.35)
  Top 0.152: 54.66,190.5 54.66,192.94 JP22.4 54.66,193.09 54.66,195.53 JP22.5 54.66,195.68 54.66,198.12 JP22.6 | 54.66,190.5 54.66,188.06 JP22.2 54.66,187.91 54.66,185.47 JP22.1 54.66,185.32 v54.66,113.39 | 54.66,190.5 JP22.3 | v73.41,83.52 73.41,108.2 (B5).10 72.34,109.27 v72.34,113.39
  Bottom 0.152: (C4).4 105.87,83.36 73.56,83.36 v73.41,83.52 | v72.34,113.39 v54.66,113.39
/128V  (via drill 0.35)
  Top 0.152: JP46.6 JP46.5 JP46.4 JP46.3 JP46.2 JP46.1 113.03,185.32 118.97,179.38 v118.97,110.8 | v108.91,91.44 108.91,107.59 110.44,109.12 (C5).10
  Bottom 0.152: v108.91,91.44 109.22,91.14 151.44,91.14 (D4).8 | v118.97,110.8 112.12,110.8 110.59,109.27 (C5).10
/256H  (via drill 0.35)
  Top 0.152: 58.47,190.5 58.47,192.94 JP23.4 58.47,193.09 58.47,195.53 JP23.5 58.47,195.68 58.47,198.12 JP23.6 | v58.47,41.76 v58.47,102.72 58.47,185.32 JP23.1 58.47,185.47 58.47,187.91 JP23.2 58.47,188.06 58.47,190.5 | 58.47,190.5 JP23.3
  Bottom 0.152: v58.47,102.72 61.06,102.72 62.13,101.65 (B5).1 | (E2).6 189.84,38.71 189.84,41.76 v58.47,41.76
/256V  (via drill 0.35)
  Top 0.152: JP47.6 JP47.5 JP47.4 JP47.3 JP47.2 JP47.1 116.84,185.32 119.58,182.57 v119.58,107.59 | (C3).2 102.97,59.74 104.5,61.27 104.5,83.52 109.52,88.54 109.52,105.61 113.03,109.12 (C5).9
  Bottom 0.152: v119.58,107.59 114.55,107.59 113.03,109.12 (C5).9
/CLK  (via drill 0.35)
  Top 0.152: 24.18,190.5 24.18,192.94 JP14.4 24.18,193.09 24.18,195.53 JP14.5 24.18,195.68 24.18,198.12 JP14.6 | v147.78,93.27 147.78,89.76 148.54,89 (D4).10 | v24.03,93.27 24.03,185.32 JP14.1 24.18,185.47 24.18,187.91 JP14.2 24.18,188.06 24.18,190.5 | 24.18,190.5 JP14.3
  Bottom 0.152: v24.03,93.27 v147.78,93.27
/COIN
  Top 0.152: (F6).2 214.99,121.01 214.99,102.56 215.9,101.65 (F5).2
  Bottom 0.152: (E5).2 180.7,99.97 214.38,99.97 | 214.38,99.97 215.9,101.5 (F5).2 215.9,101.65 218.34,101.65 (F5).3 | D1.C 230.23,99.97 214.38,99.97
/GAME  (via drill 0.35)
  Top 0.152: 175.36,217.17 175.36,219.61 JP59.5 175.36,219.76 175.36,222.2 JP59.6 | v174.14,120.24 174.45,120.55 174.45,208.79 175.21,209.55 JP59.1 175.36,209.55 175.36,211.99 JP59.2 175.36,212.14 175.36,214.58 JP59.3 175.36,214.73 175.36,217.17 | 175.36,217.17 JP59.4
  Bottom 0.152: (E6).6 187.55,120.24 v174.14,120.24
/HBLANK  (via drill 0.35)
  Top 0.152: (A3).6 38.2,59.74 38.2,67.21 (A3).9 | JP25.1 66.09,185.47 66.09,187.91 JP25.2 66.09,188.06 66.09,190.5 | 66.09,190.5 66.09,192.94 JP25.4 66.09,193.09 66.09,195.53 JP25.5 66.09,195.68 66.09,198.12 JP25.6 | 66.09,190.5 JP25.3 | v55.58,184.1 v55.58,68.89
  Bottom 0.152: v55.58,68.89 39.73,68.89 38.2,67.36 (A3).9 | v55.58,184.1 64.72,184.1 JP25.1
/HRESET  (via drill 0.35)
  Top 0.152: JP24.1 62.28,185.47 62.28,187.91 JP24.2 62.28,188.06 62.28,190.5 | 62.28,190.5 62.28,192.94 JP24.4 62.28,193.09 62.28,195.53 JP24.5 62.28,195.68 62.28,198.12 JP24.6 | 62.28,190.5 JP24.3 | v148.69,50.44 148.69,59.59 (D3).5 | v59.54,67.97 v59.54,184.71
  Bottom 0.152: (A3).10 37.74,69.49 58.01,69.49 v59.54,67.97 65.63,61.87 146.41,61.87 (D3).5 | v148.69,50.44 171.86,50.44 173.69,48.62 183.74,48.62 186.64,45.72 (E2).10 | JP24.1 61.52,184.71 v59.54,184.71
/HSYNC  (via drill 0.35)
  Top 0.152: 69.9,190.5 69.9,192.94 JP26.4 69.9,193.09 69.9,195.53 JP26.5 69.9,195.68 69.9,198.12 JP26.6 | 69.9,190.5 69.9,188.06 JP26.2 69.9,187.91 69.9,185.47 JP26.1 69.9,185.32 70.81,184.4 v70.81,124.21 | 69.9,190.5 JP26.3 | (A1).3 31.8,17.83 31.8,65.99 33.02,67.21 (A3).11 33.02,67.36 35.92,70.26 v35.92,124.21
  Bottom 0.152: (B1).2 63.19,14.94 32.11,14.94 30.58,16.46 (A1).3 | v35.92,124.21 v70.81,124.21
/START  (via drill 0.35)
  Top 0.152: 167.74,217.17 167.74,219.61 JP57.5 167.74,219.76 167.74,222.2 JP57.6 | 167.74,217.17 167.74,214.73 JP57.3 167.74,214.58 167.74,212.14 JP57.2 167.74,211.99 167.74,209.55 JP57.1 167.59,209.55 166.37,208.33 v166.37,131.22 | 167.74,217.17 JP57.4 | 177.5,122.83 176.58,121.92 (E6).1 | 177.5,122.83 177.5,131.06 v177.65,131.22 | v177.65,103.78 177.5,103.94 177.5,122.83
  Bottom 0.152: (E6).8 191.67,129.54 189.99,131.22 v177.65,131.22 v166.37,131.22 | v177.65,103.78 150.82,103.78 148.69,101.65 (D5).2
/VBLANK  (via drill 0.35)
  Top 0.152: JP49.6 JP49.5 JP49.4 JP49.3 JP49.2 JP49.1 v124.46,35.81
  Bottom 0.152: (A2).1 27.08,36.42 33.78,36.42 | 33.78,36.42 35.46,38.1 (A2).5 | 33.78,36.42 34.39,35.81 v124.46,35.81
/VRESET  (via drill 0.35)
  Top 0.152: JP48.6 JP48.5 JP48.4 JP48.3 JP48.2 JP48.1 v120.65,68.89 | v72.49,65.38 72.49,59.74 (B3).5
  Bottom 0.152: v72.49,65.38 72.8,65.68 101.3,65.68 102.82,67.21 (C3).13 102.97,67.36 104.5,68.89 v120.65,68.89
/VSYNC  (via drill 0.35)
  Top 0.152: JP50.1 JP50.2 JP50.3 JP50.4 JP50.5 JP50.6 | 30.73,87.94 31.65,88.85 (A4).12 | 30.73,87.94 30.73,69.04 31.5,68.28 31.5,22.71 25.4,16.61 (A1).1 | v32.87,188.98 32.87,124.97 30.73,122.83 30.73,87.94
  Bottom 0.152: (A1).1 25.4,16.46 27.23,14.63 64.87,14.63 65.79,15.54 65.79,17.68 65.63,17.68 65.18,18.14 63.81,18.14 62.28,16.61 (B1).1 | v32.87,188.98 127.36,188.98 128.27,188.06 JP50.2
A  (via drill 0.35)
  Top 0.152: v145.8,135.03 145.8,148.9 144.88,149.81 (D7).13
  Bottom 0.152: v145.8,135.03 146.1,134.72 187.1,134.72 188.47,136.09 207.52,136.09 210.41,138.99 253.24,138.99 256.44,142.19 (G7).3
ADDPOINT  (via drill 0.35)
  Top 0.152: JP62.1 195.63,209.55 195.63,211.99 JP62.2 195.63,212.14 195.63,214.58 JP62.3 195.63,214.73 195.63,217.17 | 195.63,217.17 195.63,219.61 JP62.5 195.63,219.76 195.63,222.2 JP62.6 | 195.63,217.17 JP62.4 | 98.25,129.23 v97.94,129.54 | v98.25,103.63 98.25,129.23 | v98.86,212.9 98.86,164.74 98.25,164.13 98.25,129.23
  Bottom 0.152: (C5).5 110.44,101.65 108,101.65 (C5).4 107.85,101.65 106.32,103.17 98.7,103.17 v98.25,103.63 | v97.94,129.54 (C6).14 | v98.86,212.9 99.16,213.21 194.41,213.21 195.48,212.14 JP62.2
ADDTENS  (via drill 0.35)
  Top 0.152: v113.94,127.25 113.94,102.56 113.03,101.65 (C5).6
  Bottom 0.152: (A6).2 34.85,127.56 60.15,127.56 | 60.15,127.56 62.13,129.54 (B6).14 | v113.94,127.25 60.45,127.25 60.15,127.56
ANTENNA  (via drill 0.35)
  Top 0.152: D5.C T1.B 188.32,178.16 188.32,162.31 190.14,160.48 v190.14,96.32 | v9.86,96.32 9.86,85.34 7.11,82.6 5.59,82.6 P1.20
  Bottom 0.152: v9.86,96.32 v190.14,96.32
B  (via drill 0.35)
  Top 0.152: v148.23,168.55 148.23,150.88 147.32,149.96 (D7).12 | v193.04,159.56 v193.04,169.32
  Bottom 0.152: v148.23,168.55 170.33,168.55 170.79,169.01 192.73,169.01 v193.04,169.32 | v193.04,159.56 193.19,159.72 256.44,159.72 257.05,160.32 257.05,162.46 256.59,162.46 (G8).3
BLUE  (via drill 0.35)
  Top 0.152: v262.53,112.17 262.53,126.19 259.18,129.54 (G6).11 | v9.86,112.17 9.86,105.16 7.11,102.41 5.59,102.41 | 5.59,102.41 v5.59,103.94 | 5.59,102.41 P1.S
  Bottom 0.152: v9.86,112.17 v262.53,112.17 | v5.59,103.94 5.59,102.41 P1.S
C
  Bottom 0.152: (D7).11 151.74,147.98 168.5,147.98 175.82,140.66 192.13,140.66 192.28,140.82 209.96,140.82 213,143.87 249.88,143.87 251.41,142.34 (G7).1
CLK  (via drill 0.35)
  Top 0.152: (E1).14 176.58,24.23 181.61,29.26 (E2).3 v181.61,43.43 | 24.18,217.17 24.18,219.61 JP1.5 24.18,219.76 24.18,222.2 JP1.6 | 24.18,217.17 24.18,214.73 JP1.3 24.18,214.58 24.18,212.14 JP1.2 24.18,211.99 24.18,209.55 JP1.1 24.03,209.55 23.11,208.64 v23.11,93.88 | 24.18,217.17 JP1.4 | 144.42,60.66 144.73,60.96 144.73,87.63 145.95,88.85 (D4).11 145.95,89 v145.95,93.88 | 144.42,60.66 143.51,59.74 (D3).3 | 144.42,60.66 v144.42,43.43
  Bottom 0.152: v145.95,93.88 v23.11,93.88 | v144.42,43.43 v181.61,43.43
COIN1  (via drill 0.35)
  Top 0.152: v5.59,131.67 5.59,130.15 P1.J 5.59,130 8.18,127.41 9.86,127.41 v9.86,115.67 | 214.68,217.17 214.68,219.61 JP67.5 214.68,219.76 214.68,222.2 JP67.6 | 214.68,217.17 214.68,214.73 JP67.3 214.68,214.58 214.68,212.14 JP67.2 214.68,211.99 214.68,209.55 JP67.1 214.53,209.55 211.02,206.05 211.02,115.67 212.24,114.45 v212.24,114.3 | 214.68,217.17 JP67.4 | v219.41,83.21 219.71,83.52 219.71,107.9 220.93,109.12 (F5).11 220.93,109.27 220.93,114.3 R10.2
  Bottom 0.152: v5.59,131.67 5.59,130.15 P1.J | (F4).1 215.29,83.21 v219.41,83.21 | R10.2 212.4,114.3 | v9.86,115.67 10.16,115.37 211.33,115.37 212.4,114.3 | 212.4,114.3 v212.24,114.3
COIN2  (via drill 0.35)
  Top 0.152: 216.81,108.2 215.9,109.12 (F5).13 | 216.81,108.2 216.97,108.05 216.97,87.94 216.2,87.17 216.2,81.69 215.9,81.38 (F4).2 | v5.59,127.71 5.59,126.19 P1.K | 218.49,217.17 218.49,219.61 JP68.5 218.49,219.76 218.49,222.2 JP68.6 | v214.99,167.64 214.99,206.2 218.34,209.55 JP68.1 218.49,209.55 218.49,211.99 JP68.2 218.49,212.14 218.49,214.58 JP68.3 218.49,214.73 218.49,217.17 | 218.49,217.17 JP68.4 | v180.7,132.28 180.7,160.17 181.31,160.78 181.31,165.66 181,165.96 181,167.03 R9.2 | v216.81,126.64 216.81,108.2
  Bottom 0.152: P1.K 5.59,126.19 v5.59,127.71 6.66,128.78 23.88,128.78 28.6,133.5 174.75,133.5 175.97,132.28 v180.7,132.28 191.06,132.28 196.39,126.95 216.51,126.95 v216.81,126.64 | R9.2 182.68,166.57 197.46,166.57 198.98,165.05 212.4,165.05 v214.99,167.64
D
  Bottom 0.152: (E7).1 170.48,148.28 154.03,148.28 152.5,149.81 (D7).10
E  (via drill 0.35)
  Top 0.152: v173.53,159.41 v173.53,149.96
  Bottom 0.152: v173.53,149.96 154.94,149.96 (D7).9 | v173.53,159.41 191.97,159.41 193.5,160.93 216.2,160.93 217.42,162.15 217.42,163.68 217.58,163.68 220.93,167.03 261.01,167.03 (G8).9
ENONES  (via drill 0.35)
  Top 0.152: (C7).12 105.41,149.81 107.85,147.37 107.85,142.34 (C7).4 | (A6).10 38.51,131.22 40.34,131.22 40.34,112.17 38.35,110.19 38.35,102.56 39.27,101.65 (A5).6 | v100.23,132.89 100.23,142.19 (C7).1
  Bottom 0.152: (C7).1 101.91,140.66 106.32,140.66 107.85,142.19 (C7).4 | (C7).9 113.03,149.96 111.51,151.49 106.93,151.49 105.41,149.96 (C7).12 | v100.23,132.89 99.92,132.59 38.2,132.59 36.83,131.22 (A6).10
ENTENS  (via drill 0.35)
  Top 0.152: (B7).12 67.31,149.81 69.75,147.37 69.75,142.34 (B7).4 | (A5).3 33.33,103.17 33.33,123.6 39.27,129.54 (A6).9 | v62.13,131.52 62.13,142.19 (B7).1
  Bottom 0.152: (B7).4 68.22,143.87 63.81,143.87 62.28,142.34 (B7).1 | (B7).9 74.93,149.96 73.41,151.49 68.83,151.49 67.31,149.96 (B7).12 | v62.13,131.52 61.82,131.22 41.1,131.22 39.42,129.54 (A6).9
F  (via drill 0.35)
  Top 0.152: v140.61,119.63 140.61,148.9 139.7,149.81 (D7).15 | v252.48,119.79 252.48,161.54 (G8).1
  Bottom 0.152: v140.61,119.63 252.32,119.63 v252.48,119.79
FIRE  (via drill 0.35)
  Top 0.152: JP69.1 222.3,209.55 222.3,211.99 JP69.2 222.3,212.14 222.3,214.58 JP69.3 222.3,214.73 222.3,217.17 | 222.3,217.17 222.3,219.61 JP69.5 222.3,219.76 222.3,222.2 JP69.6 | 222.3,217.17 JP69.4 | v15.49,122.23 v15.49,211.07 | v5.59,123.75 5.59,122.23 P1.L
  Bottom 0.152: JP69.2 221.23,211.07 v15.49,211.07 | 5.59,122.23 v15.49,122.23 | 5.59,122.23 v5.59,123.75 | 5.59,122.23 P1.L
FREIGHTER  (via drill 0.35)
  Top 0.152: v264.06,119.94 264.06,110.49 (G5).9 | JP53.1 152.5,209.55 152.5,211.99 JP53.2 152.5,212.14 152.5,214.58 JP53.3 152.5,214.73 152.5,217.17 | 152.5,217.17 152.5,219.61 JP53.5 152.5,219.76 152.5,222.2 JP53.6 | 152.5,217.17 JP53.4 | R17.2 196.85,132.13 195.48,133.5 195.48,148.44 196.85,149.81 R11.2 v196.85,207.87
  Bottom 0.152: v264.06,119.94 253.54,119.94 251.56,121.92 (G6).1 251.41,121.92 246.07,127.25 201.57,127.25 196.85,131.98 R17.2 | v196.85,207.87 154.18,207.87 152.5,209.55 JP53.1
G  (via drill 0.35)
  Top 0.152: v193.8,148.44 v193.8,140.21
  Bottom 0.152: (D7).14 148.23,143.87 172.16,143.87 175.82,140.21 v193.8,140.21 | v193.8,148.44 212.85,148.44 213,148.28 247.9,148.28 251.1,151.49 262.53,151.49 (G7).9
GAME  (via drill 0.35)
  Top 0.152: 171.55,209.55 171.55,211.99 JP58.2 171.55,212.14 171.55,214.58 JP58.3 171.55,214.73 171.55,217.17 | 171.55,217.17 171.55,219.61 JP58.5 171.55,219.76 171.55,222.2 JP58.6 | 171.55,217.17 JP58.4 | (F7).11 220.93,149.96 220.93,151.49 218.03,151.49 217.42,150.88 217.42,143.26 (F7).3 218.34,142.19 218.34,131.37 217.42,130.45 v217.42,123.6 | (E5).4 185.72,103.17 185.72,121.01 186.64,121.92 (E6).5 | 171.55,209.55 172.62,208.48 v172.62,124.21 | 171.55,209.55 JP58.1
  Bottom 0.152: 188.47,123.6 v217.42,123.6 | 188.47,123.6 186.79,121.92 (E6).5 | v172.62,124.21 172.92,123.9 188.16,123.9 188.47,123.6
GND
  Top 0.152: R9.1 171.4,167.64 171.4,170.08 R29.1 | T1.E 186.79,179.07 186.79,172.82 T2.E 186.64,172.67 186.64,160.32 183.9,160.32 182.98,161.24 C6.2 | C7.2 237.39,186.69 229.62,178.92 229.62,163.37 229.01,162.76 (F8).7 | 207.06,144.78 207.06,147.22 R12.1 207.06,147.37 207.06,149.81 R11.1 | 207.06,137.16 207.06,134.72 R16.1 207.06,134.57 207.06,132.13 R17.1 207.06,131.98 207.06,117.96 210.72,114.3 R10.1 | 207.06,137.16 207.06,139.6 R15.1 207.06,139.75 207.06,142.19 R14.1 207.06,142.34 207.06,144.78 | 207.06,137.16 R5.2 | 207.06,144.78 R13.1
  Top 1.016: (A8).7 41.91,153.66 43.23,152.34 43.23,149.92 41.91,148.6 (A7).7 41.91,132.07 43.23,130.75 43.23,128.33 41.91,127.01 (A6).7 41.91,111.75 43.23,110.43 43.23,108.01 41.91,106.69 (A5).7 41.91,91.43 43.23,90.11 43.23,87.69 41.91,86.37 (A4).7 41.91,68.57 41.96,68.52 41.96,61.01 (A3).7 40.64,48.25 41.96,46.93 41.96,44.51 40.64,43.19 (A2).7 40.64,26.66 41.96,25.34 41.96,22.92 40.64,21.6 (A1).7 40.64,3.17 | (B7).7 77.47,132.07 78.79,130.75 78.79,108.01 77.47,106.69 (B5).7 77.47,91.43 78.79,90.11 78.79,87.69 77.47,86.37 (B4).7 77.47,69.84 78.79,68.52 78.79,66.1 77.47,64.78 (B3).7 77.47,48.25 78.79,46.93 78.79,44.51 77.47,43.19 (B2).7 77.47,26.66 78.79,25.34 78.79,22.92 77.47,21.6 (B1).7 77.47,3.17 | (B7).7 77.47,134.62 (B6).10 | (B7).7 77.47,147.33 78.79,148.65 78.79,151.07 77.47,152.39 (B8).7 | (C8).7 115.57,152.39 116.89,151.07 116.89,148.65 115.57,147.33 (C7).7 115.57,134.62 | 115.57,134.62 (C6).10 | 115.57,134.62 115.57,132.07 116.89,130.75 116.89,108.01 115.57,106.69 (C5).7 115.57,91.43 116.89,90.11 116.89,87.69 115.57,86.37 (C4).7 115.57,69.84 116.89,68.52 116.89,66.1 115.57,64.78 (C3).7 | (C3).7 115.57,50.8 (C2).10 | (C3).7 115.57,48.25 116.89,46.93 116.89,30.53 | 116.89,30.53 (C1).10 | 153.67,29.21 (D2).7 153.67,43.19 154.99,44.51 154.99,46.93 153.67,48.25 (D3).7 153.67,64.78 154.99,66.1 154.99,68.52 153.67,69.84 (D4).7 153.67,86.37 154.99,87.69 154.99,92.66 | 153.67,29.21 (D1).10 | 154.99,92.66 (D5).1 | 154.99,92.66 154.99,100.84 155.14,100.99 155.14,121.72 (D6).7 154.94,127.01 156.26,128.33 156.26,130.75 154.94,132.07 (D7).8 154.94,147.33 156.26,148.65 156.26,151.07 154.94,152.39 (D8).7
